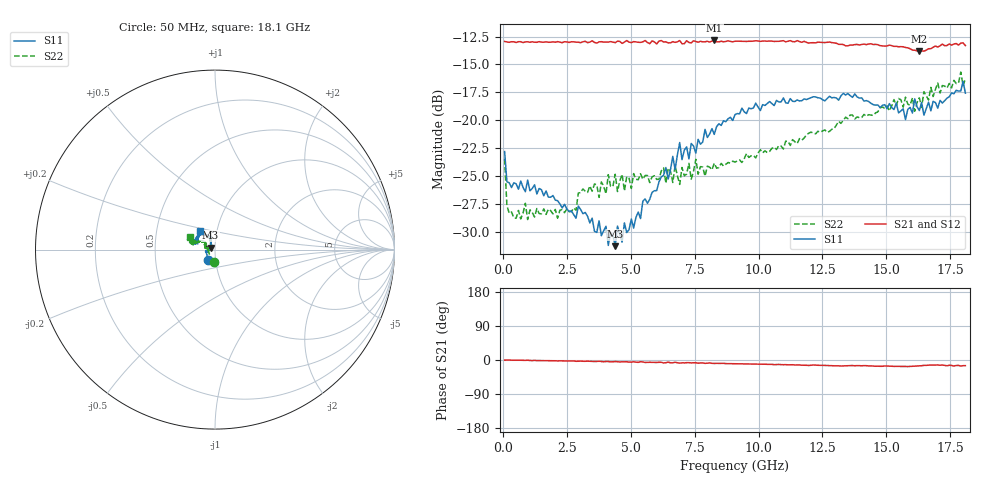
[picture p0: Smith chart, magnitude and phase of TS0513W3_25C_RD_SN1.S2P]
! Network Analyzer HP8720D.06.14 Serial No. US36140669
! 17 Jun 2005  08:17:59
! Frequency  S11  S21  S12  S22
# HZ  S  DB R 50
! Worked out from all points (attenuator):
!   201 points, 50 MHz to 18.1 GHz, reference 50 ohm
!   highest |S21| = -12.85 dB at 8.263 GHz (marker M1); lowest = -13.8 dB at 16.3 GHz (marker M2)
!   lowest |S11| = -31.3 dB at 4.382 GHz (marker M3), VSWR 1.06, Z = 47.6 + j1.09 ohm
!   |S11| at or under -10 dB: start of sweep to end of sweep
!   |S22| runs from -28.9 to -15.7 dB; largest |S21 - S12| = 0.0068
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5e7  -22.81 -125.1  -12.94 -0.3  -12.96 -0.1  -23.48 -95.1
1.4025e8  -25.52 -148.2  -12.98 -0.2  -13.00 -0.2  -27.65 -136.4
4.11e8  -25.62 -166.0  -12.97 -0.5  -12.99 -0.4  -28.75 -161.9
2.12575e9  -27.22 -169.5  -12.96 -2.4  -13.00 -2.3  -28.79 167.4
3.1185e9  -28.38 -174.5  -12.97 -3.3  -12.99 -3.4  -26.16 171.8
4.382e9  -31.29 155.0  -13.05 -4.1  -12.97 -4.6  -24.85 168.3
4.47225e9  -29.49 148.1  -12.91 -4.7  -12.98 -4.2  -26.39 171.4
4.65275e9  -30.93 141.7  -13.11 -4.9  -12.97 -4.7  -24.85 171.2
4.743e9  -29.20 144.3  -13.00 -4.7  -13.03 -4.6  -26.34 166.7
5.104e9  -29.67 135.2  -12.95 -4.8  -12.90 -5.1  -24.79 162.8
6.09675e9  -25.54 116.4  -12.91 -6.0  -12.88 -6.1  -25.30 161.3
6.7285e9  -24.43 117.6  -13.02 -5.9  -13.09 -6.7  -24.08 155.6
6.909e9  -22.00 114.7  -12.86 -8.2  -13.00 -7.8  -25.76 151.0
7.27e9  -23.47 111.7  -13.03 -7.0  -13.03 -7.9  -23.87 153.2
7.36025e9  -22.09 109.0  -13.07 -7.8  -13.03 -7.2  -25.30 155.9
7.54075e9  -22.95 110.2  -12.95 -7.3  -12.85 -8.3  -23.51 155.5
8.26275e9  -21.27 121.0  -12.85 -9.1  -12.93 -9.2  -23.86 144.2
9.075e9  -19.50 126.6  -12.92 -9.7  -12.92 -9.6  -23.75 145.5
1.21435e10  -17.90 156.8  -13.05 -13.2  -13.04 -13.4  -21.16 148.8
1.512175e10  -18.51 161.1  -13.26 -16.2  -13.25 -15.7  -19.16 161.2
1.6295e10  -19.13 148.4  -13.83 -15.7  -13.76 -15.7  -17.99 167.9
1.81e10  -17.57 130.3  -13.31 -14.8  -13.32 -16.3  -16.29 153.8
